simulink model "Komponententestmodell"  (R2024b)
settings: Solver=VariableStepAuto  StartTime=0.0  StopTime=10.0  RelTol=1e-3
libraries: arduinolib x7

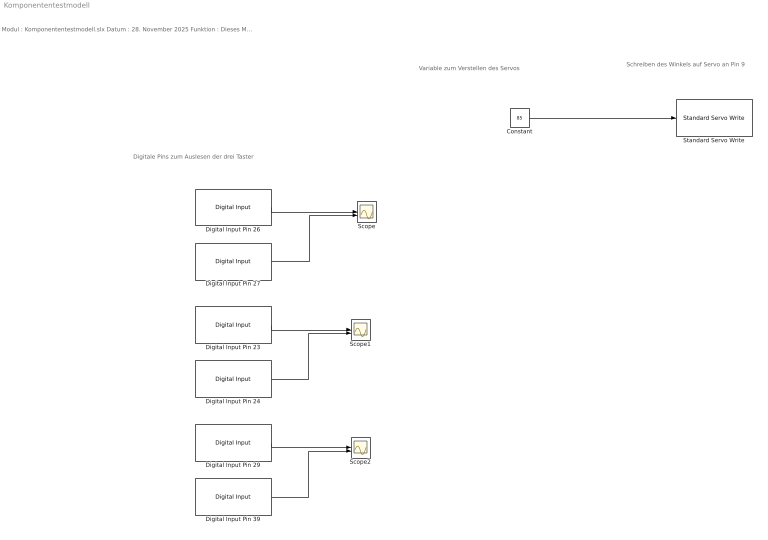
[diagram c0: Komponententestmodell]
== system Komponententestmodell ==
  note: Variable zum Verstellen des Servos
  note: Schreiben des Winkels auf Servo an Pin 9
  note: Modul : Komponententestmodell.slx Datum : 28. November 2025 Funktion : Dieses Modell wird zum Komponententest des Servos und der Kippschalter genutzt Implementierung : Simulink (R2024b) Req. Toolbox : Simulink Support Package for Arduino Hardware Autor : Kilian Engelhardt, Daniel Block Bemerkung : Getestet Letzte Änderung : 8. Dez 2025
  note: Digitale Pins zum Auslesen der drei Taster
  Constant : Constant  Value=85
  Digital Input Pin 23 : arduinolib/Digital Input  pinNumber=23  mode=Input Pullup  Direction=input  SampleTime=0.1  blockPlatform=arduino
  Digital Input Pin 24 : arduinolib/Digital Input  pinNumber=24  mode=Input Pullup  Direction=input  SampleTime=0.1  blockPlatform=arduino
  Digital Input Pin 26 : arduinolib/Digital Input  pinNumber=26  mode=Input Pullup  Direction=input  SampleTime=0.1  blockPlatform=arduino
  Digital Input Pin 27 : arduinolib/Digital Input  pinNumber=27  mode=Input Pullup  Direction=input  SampleTime=0.1  blockPlatform=arduino
  Digital Input Pin 29 : arduinolib/Digital Input  pinNumber=29  mode=Input Pullup  Direction=input  SampleTime=0.1  blockPlatform=arduino
  Digital Input Pin 39 : arduinolib/Digital Input  pinNumber=39  mode=Input Pullup  Direction=input  SampleTime=0.1  blockPlatform=arduino
  Scope : Scope  NumInputPorts=2
  Scope1 : Scope  NumInputPorts=2
  Scope2 : Scope  NumInputPorts=2
  Standard Servo Write : arduinolib/Standard Servo Write  pinNumber=9  ServoIndex=0  blockPlatform=ARDUINO
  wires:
  Constant/1 -> Standard Servo Write/1
  Digital Input Pin 39/1 -> Scope2/2
  Digital Input Pin 29/1 -> Scope2/1
  Digital Input Pin 23/1 -> Scope1/1
  Digital Input Pin 26/1 -> Scope/1
  Digital Input Pin 24/1 -> Scope1/2
  Digital Input Pin 27/1 -> Scope/2
